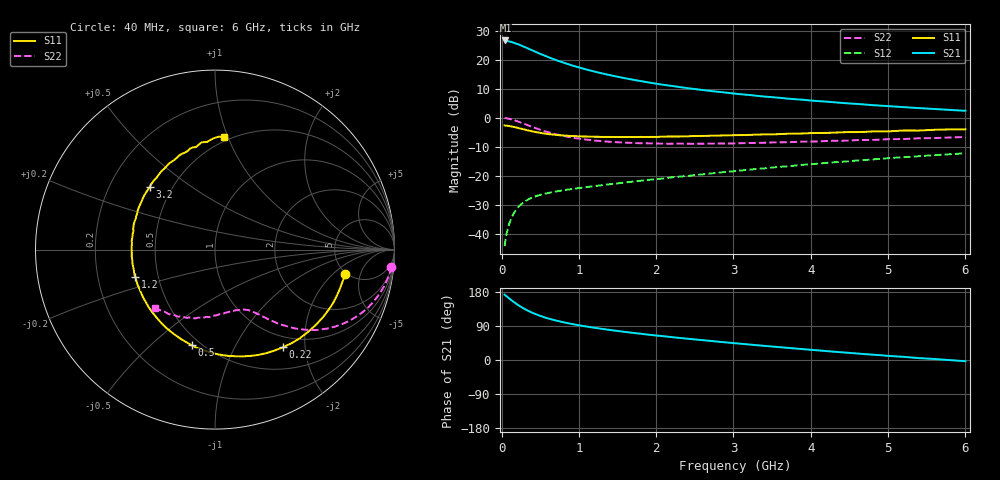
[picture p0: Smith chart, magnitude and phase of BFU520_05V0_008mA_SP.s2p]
! Filename:  P:\Prog\Test\Noise\ATS_data\Testdata_Net\03 Spar\BFU520_APG2013_37_A05_05p0V_008mA_SP_CM01_D.s2p
! Date/Time: Fri 26/Apr/2013 13:00:08
! BFU520_APG2013_37_A05_05p0V_1to20mA_SP_CM01_Bias5_R.s2p
! MDIF S-parameter v. bias file
! BFU520_APG2013_37_A05_05p0V_1to20mA_SP_CM01
! Date/time Tue Apr 23 15:26:19 2013
! VAR V_out= 5.0010
! VAR I_out= 7.9950
! VAR V_in= 0.8353
! VAR I_in= 0.0911
! Device data file deembeded for feedlines and parallel
! Original file: \03 Spar\BFU520_APG2013_37_A05_05p0V_008mA_SP_CM01_R.s2p
! Feed-files: PR047V01_250413_Feed1.s2p, PR047V01_250413_Feed2.s2p
! Parallel-file: PR047V01_250413_Par.s2p
# MHz S MA R 50
!  Freq-MHz  S11-mag  S11-arg  S21-mag  S21-arg  S12-mag  S12-arg  S22-mag  S22-arg
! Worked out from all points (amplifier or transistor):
!   98 points, 40 MHz to 6 GHz, reference 50 ohm
!   highest |S21| = 26.6 dB at 50 MHz (marker M1)
!   |S21| within 3 dB of that: start of sweep to 362.5 MHz
!   unconditionally stable (mu >= 1): 1.926 GHz to 4.084 GHz
!   at 300 MHz: K = 0.27, MSG = 26.6 dB, |S12| = -28.9 dB
!   at 1.6 GHz: K = 0.94, MSG = 18.0 dB, |S12| = -22.3 dB
!   at 6 GHz: K = 0.85, MSG = 7.3 dB, |S12| = -12.3 dB
!   S11 on the Smith chart (normalised r, x): 40 MHz: 4.82, -2.87; 220 MHz: 0.82, -1.59; 500 MHz: 0.45, -0.68; 1.2 GHz: 0.37, -0.14; 3.2 GHz: 0.38, +0.35; 6 GHz: 0.46, +0.97
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40  0.7363 -10.7  21.45 172.6  0.006112 84.6  0.9864 -5.5
50  0.7337 -13.4  21.45 170.2  0.007675 83.4  0.9845 -6.9
60  0.7305 -15.8  21.09 169.1  0.009172 82.2  0.9801 -8.3
80  0.7252 -21.2  20.94 165.7  0.01209 79.6  0.9697 -11.0
140  0.7016 -36.6  19.98 155.8  0.02018 72.5  0.9271 -18.6
220  0.6631 -55.2  18.33 144.3  0.02909 64.7  0.854 -27.2
260  0.6438 -63.8  17.41 139.2  0.03273 61.4  0.816 -30.8
320  0.6143 -75.6  16.12 132.3  0.03732 57.3  0.76 -35.5
400  0.5815 -89.2  14.44 124.5  0.04207 53.3  0.6912 -40.3
500  0.5486 -103.8  12.63 116.6  0.04677 49.8  0.621 -44.9
600  0.5234 -116.0  11.16 109.9  0.05033 47.6  0.5643 -48.2
750  0.4993 -130.8  9.384 102.0  0.05482 45.9  0.5024 -51.8
900  0.4837 -142.8  8.064 95.5  0.05874 45.3  0.4585 -54.5
1050  0.4747 -152.7  7.052 89.9  0.06244 45.4  0.4274 -56.8
1200  0.4695 -161.1  6.251 85.0  0.06616 45.8  0.405 -58.8
1600  0.4639 -179.2  4.781 74.0  0.07648 47.2  0.3719 -64.0
2050  0.4701 166.0  3.765 63.6  0.08862 48.7  0.358 -70.6
3100  0.5017 137.5  2.536 42.8  0.1232 49.6  0.3638 -87.2
3200  0.5052 135.9  2.469 41.0  0.1274 49.5  0.3663 -88.5
4100  0.546 116.4  1.931 25.3  0.1619 46.6  0.3904 -104.0
5200  0.6024 97.1  1.522 8.4  0.2088 40.4  0.429 -122.6
6000  0.631 85.3  1.317 -3.2  0.2436 34.3  0.4654 -136.0
